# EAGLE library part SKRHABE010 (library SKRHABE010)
Multi-Directional Switches 4-directn cntr push W/boss 200K Cycles Source: Datasheet
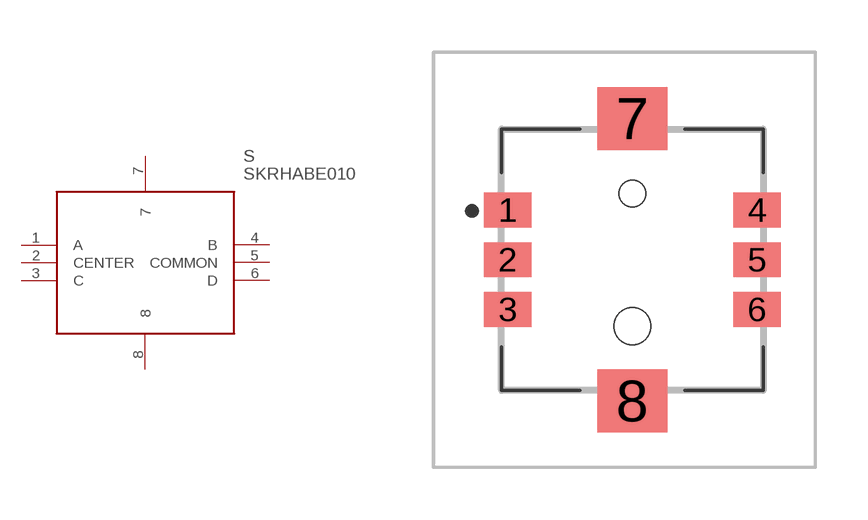
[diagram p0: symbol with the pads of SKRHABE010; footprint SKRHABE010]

Designator prefix S

## SKRHABE010 (Arrow_Part_Number: SKRHABE010; Arrow_Price-Stock: https://www.arrow.com/en/products/skrhabe010/alps-electric; Description: Multi-Directional Switches 4-directn cntr push W/boss 200K Cycles; Height: 5mm; Manufacturer_Name: ALPS Electric; Manufacturer_Part_Number: SKRHABE010; Mouser_Part_Number: 688-SKRHAB; Mouser_Price-Stock: https://www.mouser.co.uk/ProductDetail/Alps-Alpine/SKRHABE010?qs=seHrhfPpLDxEOwRqoDvYHw%3D%3D)  [SKRHABE010]
1  A
2  CENTER
3  C
4  B
5  COMMON
6  D
7  7
8  8

## Footprint SKRHABE010 (pad centres in mm)
SKRHABE010-1
smd 1.35 x 1: 1 -3.575,1.425; 2 -3.575,0; 3 -3.575,-1.425; 4 3.575,1.425; 5 3.575,0; 6 3.575,-1.425
smd 2 x 1.8: 7 0,4.05; 8 0,-4.05
hole 0.75 at 0,1.9
hole 1.05 at 0,-1.9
